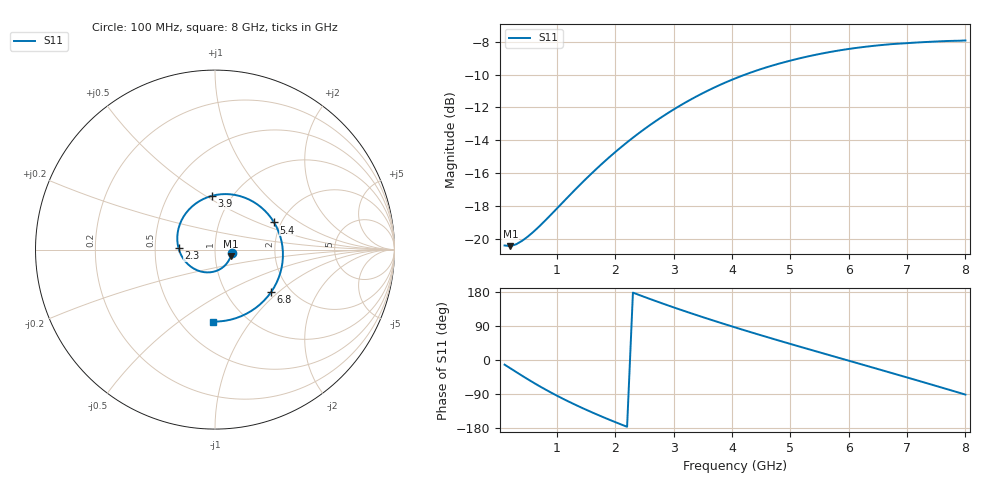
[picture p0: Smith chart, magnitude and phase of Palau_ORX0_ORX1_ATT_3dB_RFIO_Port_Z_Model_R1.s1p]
! Created Fri Oct  9 14:28:59 2020
! Palau ORX0/ORX1 RFIO Port Impedance Model.
! Attenuation  : 3 dB.
! Revision		: R1.
! Impedance Mode 	: Balanced Differential-Mode.
! Impedance Format 	: Series Equivalent Differential Impedance (SEDZ).
# hz S ma R 100
! 1 Port Network Data from SP1.SP block
! freq  magS11  angS11
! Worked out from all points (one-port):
!   80 points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, 100 MHz to 8 GHz, reference 100 ohm
!   lowest |S11| = -20.4 dB at 200 MHz (marker M1), VSWR 1.21, Z = 119 - j8.59 ohm
!   |S11| at or under -10 dB: start of sweep to 4.224 GHz
!   S11 on the Smith chart (normalised r, x): 100 MHz: 1.20, -0.05; 2.3 GHz: 0.66, +0.01; 3.9 GHz: 0.81, +0.53; 5.4 GHz: 1.84, +0.64; 6.8 GHz: 1.60, -0.90; 8 GHz: 0.71, -0.68
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1e8  0.0956 -12.3
2e8  0.09513 -22.1
4e8  0.09876 -41.5
7e8  0.1095 -69.2
1.1e9  0.1294 -102.2
1.3e9  0.1407 -117.2
1.6e9  0.1588 -138.2
1.8e9  0.1713 -151.4
2.1e9  0.1904 -170.2
2.3e9  0.2033 177.8
2.7e9  0.229 155.0
3.1e9  0.254 133.5
3.5e9  0.2778 113.0
3.9e9  0.2999 93.3
4.1e9  0.3102 83.8
4.3e9  0.3199 74.4
4.6e9  0.3332 60.5
4.8e9  0.3412 51.4
5.1e9  0.3523 37.9
5.4e9  0.3623 24.6
5.8e9  0.3736 7.0
6.1e9  0.3806 -6.2
6.4e9  0.3863 -19.4
6.8e9  0.3922 -37.2
7.1e9  0.3952 -50.5
7.4e9  0.3979 -64.0
7.6e9  0.3994 -73.1
8e9  0.4016 -91.3
